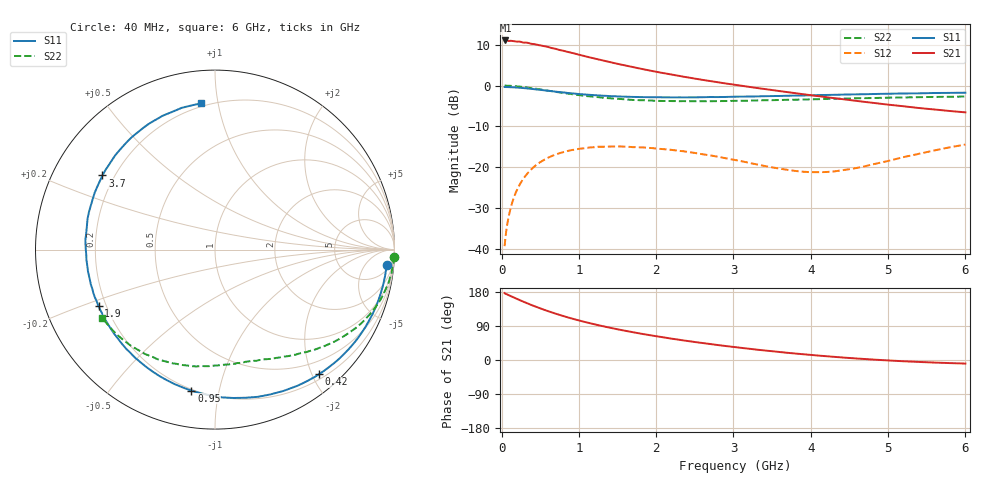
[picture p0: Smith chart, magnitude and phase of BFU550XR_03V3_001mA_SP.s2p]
! Filename:  P:\Prog\Test\Noise\ATS_data\Testdata_Net\03 Spar\BFU550XR_APG2013_45_C05_03p3V_001mA_SP_CM01_D.s2p
! Date/Time: Tue 06/Aug/2013 14:38:14
! BFU550XR_APG2013_45_C05_03p3V_1to35mA_SP_CM01_Bias1_R.s2p
! MDIF S-parameter v. bias file
! BFU550XR_APG2013_45_C05_03p3V_1to35mA_SP_CM01
! Date/time Fri Aug 02 14:41:13 2013
! bias mode 1
! bias variable = I_out
! VAR bias_var= 1
! VAR V_out= 3.3000
! VAR I_out= 1.0000
! VAR V_in= 0.7776
! VAR I_in= 0.0109
! Device data file deembeded for feedlines and parallel
! Original file: \03 Spar\BFU550XR_APG2013_45_C05_03p3V_001mA_SP_CM01_R.s2p
! Feed-files: PR006V01_02082013_Feed1.s2p, PR006V01_02082013_Feed2.s2p
! Parallel-file: PR006V01_02082013_Par.s2p
# MHz S MA R 50
!  Freq-MHz  S11-mag  S11-arg  S21-mag  S21-arg  S12-mag  S12-arg  S22-mag  S22-arg
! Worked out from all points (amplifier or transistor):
!   98 points, 40 MHz to 6 GHz, reference 50 ohm
!   highest |S21| = 11.0 dB at 50 MHz (marker M1)
!   |S21| within 3 dB of that: start of sweep to 903 MHz
!   unconditionally stable (mu >= 1): 3.427 GHz to 4.96 GHz
!   at 300 MHz: K = 0.09, MSG = 16.4 dB, |S12| = -22.3 dB
!   at 1.6 GHz: K = 0.39, MSG = 9.9 dB, |S12| = -14.9 dB
!   at 6 GHz: K = 0.82, MSG = 3.9 dB, |S12| = -14.4 dB
!   S11 on the Smith chart (normalised r, x): 40 MHz: 9, -19; 420 MHz: 0.28, -2.10; 950 MHz: 0.19, -0.83; 1.9 GHz: 0.17, -0.22; 3.7 GHz: 0.15, +0.29; 6 GHz: 0.18, +0.89
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40  0.9606 -5.0  3.548 176.6  0.01092 86.9  0.9982 -2.2
50  0.9599 -6.2  3.556 174.7  0.01364 86.3  0.9988 -3.0
100  0.9567 -12.5  3.503 170.5  0.0271 81.9  0.9931 -6.4
120  0.9548 -15.0  3.526 168.6  0.03241 80.3  0.9921 -7.7
180  0.9484 -22.3  3.461 163.1  0.04806 75.5  0.9824 -11.5
320  0.9245 -39.0  3.35 150.7  0.08115 65.1  0.95 -19.8
420  0.904 -50.2  3.211 142.5  0.1017 58.4  0.9218 -25.1
600  0.8638 -69.1  2.968 129.0  0.1309 47.2  0.8666 -33.7
800  0.8242 -87.4  2.662 116.0  0.154 36.8  0.8115 -41.6
950  0.797 -99.5  2.456 107.2  0.1653 30.0  0.7743 -46.8
1050  0.7821 -106.9  2.32 101.8  0.1706 26.1  0.753 -49.8
1250  0.758 -120.3  2.088 92.0  0.1788 18.9  0.7224 -55.1
1450  0.7415 -132.0  1.889 83.2  0.1802 12.6  0.6939 -60.4
1700  0.7266 -145.0  1.683 73.3  0.177 6.0  0.6669 -66.5
1900  0.7214 -154.1  1.538 66.2  0.1732 1.4  0.6559 -70.8
2050  0.7195 -160.4  1.444 61.2  0.1685 -1.4  0.6491 -73.9
2500  0.7177 -177.4  1.216 47.5  0.1503 -8.2  0.6443 -83.0
3100  0.7329 163.3  0.9963 32.1  0.1192 -10.1  0.6518 -94.9
3700  0.751 146.6  0.8315 19.0  0.09345 -0.8  0.6699 -106.6
4100  0.7651 136.5  0.7424 11.6  0.08743 13.2  0.6819 -114.2
5200  0.8007 111.4  0.5587 -3.3  0.1337 39.8  0.7156 -134.6
6000  0.8182 95.4  0.4708 -9.4  0.1904 39.3  0.7344 -148.8
